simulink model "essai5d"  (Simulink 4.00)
settings: Solver=ode45  SolverMode=SingleTasking  StartTime=0.0  StopTime=tend*2  FixedStep=[]  MaxStep=1  RelTol=1e-3  AbsTol=1e-3
PreLoadFcn:
  | demo2dat
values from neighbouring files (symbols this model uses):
  delt = 0.2    [demo1dat.m]    (also in essai1dat.m; essai2dat.m = 0.1)
  m = 4    [demo1dat.m]    (also in demo2dat.m = 3; essai1dat.m; essai2dat.m = 6; mynlcmpc.m = mp(1:max(size(mp))-1))
  model = tfd2step(1.6,delt,1,g)    [essai2dat.m]    (also in mynlcmpc.m = modelpd(:,1:nu); mynlcmpc2.m = modelpd(:,1:nu); mynlcmpc3.m = modelpd(:,1:nu); scrtp1.m = tfd2step(tfinal,Ts,1,g))
  p = 10    [demo1dat.m]    (also in demo2dat.m; essai1dat.m; essai2dat.m; mynlcmpc.m = mp(max(size(mp))))
  ulim = [-5 40 3]    [essai2dat.m]    (also in mynlcmpc.m = [-inf*ones(1,nu) inf*ones(1,nu) 1e6*ones(1,nu)]; mynlcmpc2.m = [-inf*ones(1,nu) inf*ones(1,nu) 1e6*ones(1,nu)]; mynlcmpc3.m = [-inf*ones(1,nu) inf*ones(1,nu) 1e6*ones(1,nu)]; pmlin.m = [-10*[1 1] 10*[1 1] 2*[1 1]])
  uwt = [0 0]    [demo1dat.m]    (also in demo2dat.m = 0.6*[1 1]; essai1dat.m; essai2dat.m = 1; mynlcmpc.m = ryuwt(:,2*ny+1:2*ny+nu))
  ylim = [-40 40]    [essai2dat.m]    (also in mynlcmpc.m = [ylim; ylim(N,:)]; mynlcmpc2.m = [ylim; ylim(N,:)]; mynlcmpc3.m = [ylim; ylim(N,:)]; pmlin.m = [])
  ywt = [1 1]    [demo1dat.m]    (also in demo2dat.m = [0.2,0,1]; essai1dat.m; essai2dat.m = 1; mynlcmpc.m = ryuwt(:,ny+1:2*ny))

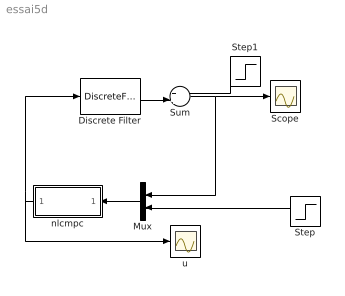
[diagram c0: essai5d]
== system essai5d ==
  Discrete Filter : DiscreteFilter  Numerator="[ 0  0  1]"  Denominator=[1 0.5]  SampleTime=delt  Realization=auto
  Mux : Mux  Orientation=left  Inputs=2
  Scope : Scope
  Step : Step  Orientation=left  Time=0  Before=0  After=10  SampleTime=0
  Step1 : Step  Orientation=left  Time=2  Before=0  After=-3  SampleTime=0
  Sum : Sum  Inputs=++|  SaturateOnIntegerOverflow=on
  nlcmpc : Subsystem  Orientation=left  AncestorBlock=nlmpclib/nlcmpc  mask(myCMPC-SIMULINK){modelpd=[model []], yuwt=[ywt uwt], mp=[m p], yulim=[ylim ulim], tfilter=[], ud0=[0 []]}
      mask help: Masked MATLAB function block calls nlcmpc, links CMPC and SIMULINK.
  u : Scope
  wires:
  nlcmpc/1(Out1) -> u/1, Discrete Filter/1
  Mux/1 -> nlcmpc/1(In1)
  Step/1 -> Mux/2
  Discrete Filter/1 -> Sum/2
  Sum/1 -> Scope/1, Mux/1
  Step1/1 -> Sum/1

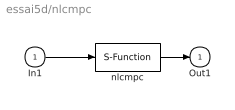
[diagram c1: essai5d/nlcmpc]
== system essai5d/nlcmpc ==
  In1 : Inport  Port=1  LatchInput=off
  nlcmpc : S-Function  FunctionName=mynlcmpc3  Parameters=modelpd,mp,tfilter,yuwt,ud0,yulim  PortCounts=[]  SFunctionModules=''
  Out1 : Outport  Port=1  InitialOutput=0
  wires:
  In1/1 -> nlcmpc/1
  nlcmpc/1 -> Out1/1
